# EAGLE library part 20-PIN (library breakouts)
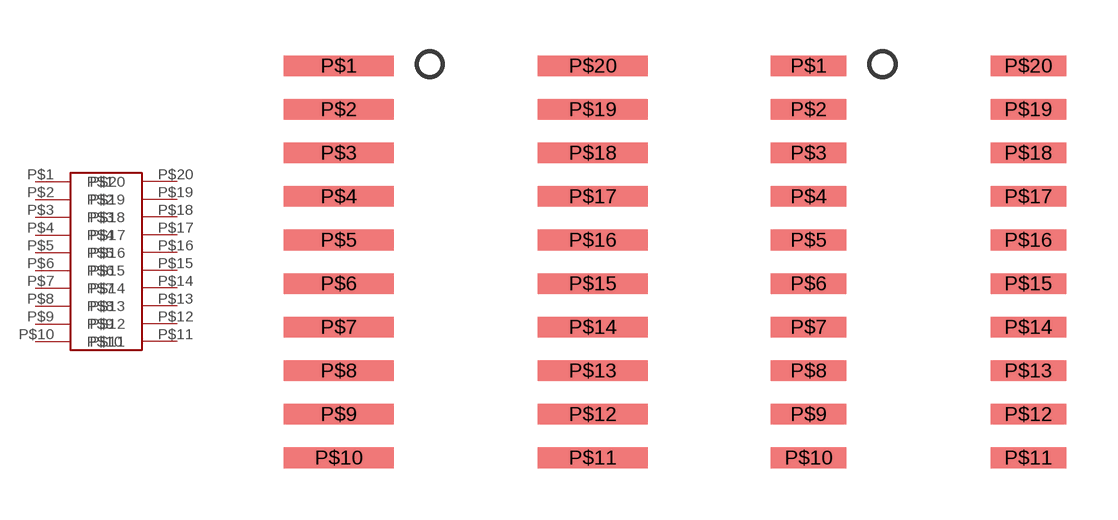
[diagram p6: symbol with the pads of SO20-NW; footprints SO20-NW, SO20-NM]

Designator prefix -

## 20-PINSOIC-NW  [SO20-NW]
P$1  P$1
P$2  P$2
P$3  P$3
P$4  P$4
P$5  P$5
P$6  P$6
P$7  P$7
P$8  P$8
P$9  P$9
P$10  P$10
P$11  P$11
P$12  P$12
P$13  P$13
P$14  P$14
P$15  P$15
P$16  P$16
P$17  P$17
P$18  P$18
P$19  P$19
P$20  P$20

## 20-PINSOIC-NM  [SO20-NM]
Pads as for SO20-NW

## 20-PINSOIC-M  [SO20-M]
Pads as for SO20-NW

## 20-PINTSSOP-N  [TSSOP20-3.9]
Pads as for SO20-NW

## 20-PINSOIC-N  [SO20-N]
Pads as for SO20-NW

## 20-PINSOIC-MW  [SO20-MW]
Pads as for SO20-NW

## 20-PINSOIC-W  [SO20-W]
Pads as for SO20-NW

## 20-PINTSSOP-W  [TSSOP20-5.3]
Pads as for SO20-NW

## 20-PINTSSOP-NW  [TSSOP20-NW]
Pads as for SO20-NW

## Footprint SO20-NW (pad centres in mm)
smd 3.2 x 0.6: P$1 -3.7,5.715; P$2 -3.7,4.445; P$3 -3.7,3.175; P$4 -3.7,1.905; P$5 -3.7,0.635; P$6 -3.7,-0.635; P$7 -3.7,-1.905; P$8 -3.7,-3.175; P$9 -3.7,-4.445; P$10 -3.7,-5.715; P$11 3.7,-5.715; P$12 3.7,-4.445; P$13 3.7,-3.175; P$14 3.7,-1.905; P$15 3.7,-0.635; P$16 3.7,0.635; P$17 3.7,1.905; P$18 3.7,3.175; P$19 3.7,4.445; P$20 3.7,5.715

## Footprint SO20-NM (pad centres in mm)
smd 2.2 x 0.6: P$1 -3.2,5.715; P$2 -3.2,4.445; P$3 -3.2,3.175; P$4 -3.2,1.905; P$5 -3.2,0.635; P$6 -3.2,-0.635; P$7 -3.2,-1.905; P$8 -3.2,-3.175; P$9 -3.2,-4.445; P$10 -3.2,-5.715; P$11 3.2,-5.715; P$12 3.2,-4.445; P$13 3.2,-3.175; P$14 3.2,-1.905; P$15 3.2,-0.635; P$16 3.2,0.635; P$17 3.2,1.905; P$18 3.2,3.175; P$19 3.2,4.445; P$20 3.2,5.715

## Footprint SO20-M (pad centres in mm)
smd 1.2 x 0.6: P$1 -3.7,5.715; P$2 -3.7,4.445; P$3 -3.7,3.175; P$4 -3.7,1.905; P$5 -3.7,0.635; P$6 -3.7,-0.635; P$7 -3.7,-1.905; P$8 -3.7,-3.175; P$9 -3.7,-4.445; P$10 -3.7,-5.715; P$11 3.7,-5.715; P$12 3.7,-4.445; P$13 3.7,-3.175; P$14 3.7,-1.905; P$15 3.7,-0.635; P$16 3.7,0.635; P$17 3.7,1.905; P$18 3.7,3.175; P$19 3.7,4.445; P$20 3.7,5.715

## Footprint TSSOP20-3.9 (pad centres in mm)
smd 1.4 x 0.35: P$1 -2.65,2.925; P$2 -2.65,2.275; P$3 -2.65,1.625; P$4 -2.65,0.975; P$5 -2.65,0.325; P$6 -2.65,-0.325; P$7 -2.65,-0.975; P$8 -2.65,-1.625; P$9 -2.65,-2.275; P$10 -2.65,-2.925; P$11 2.65,-2.925; P$12 2.65,-2.275; P$13 2.65,-1.625; P$14 2.65,-0.975; P$15 2.65,-0.325; P$16 2.65,0.325; P$17 2.65,0.975; P$18 2.65,1.625; P$19 2.65,2.275; P$20 2.65,2.925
